FUNCTION_BLOCK FB_EL5131_SingleCycle
VAR_INPUT PERSISTENT
	arDataSingle											:	ARRAY[1..2] OF ST_EL5131_CamData;
END_VAR
VAR_INPUT
	bSetCounter												:	BOOL;
	nSetCounterValue										:	UDINT;
	bReset													:	BOOL;
	bRun													:	BOOL;
	stEl5131												:	REFERENCE TO ST_EL5131;
END_VAR
VAR_OUTPUT
	bInited													:	BOOL;
END_VAR
VAR
	{attribute 'hide'}
	_bLastCounterValue										:	BOOL;
	{attribute 'hide'}
	nLastCounterValue										:	UDINT;
	{attribute 'hide'}
	bForward												:	BOOL;
	{attribute 'hide'}
	bBackward												:	BOOL;
	{attribute 'hide'}
	rtSetCounter											:	R_TRIG;
END_VAR


// check REFERENCE
IF NOT __ISVALIDREF(stEl5131)
THEN 
	RETURN;
END_IF

// reset
IF bReset THEN 
	stEl5131.PlcToPdo.Contro_OutputChn1.Control.Enable_thresholds_output		:= FALSE;
	bReset 																		:= FALSE;	
	bInited																		:= FALSE;
END_IF

// init
IF NOT bInited THEN 
	stEl5131.PlcToPdo.Contro_OutputChn1.Control.Enable_thresholds_output		:= TRUE;
	stEl5131.PlcToPdo.Contro_OutputChn1.Control.Disalbe_thresholds_ccw			:= TRUE; // 在RUN 中根据情况再给false
	stEl5131.PlcToPdo.Contro_OutputChn1.Control.Disalbe_thresholds_cw			:= TRUE; // 在RUN 中根据情况再给false
	stEl5131.PlcToPdo.Contro_OutputChn1.Control.Set_tristate					:= FALSE;
	bInited																		:= TRUE;
END_IF

// set counter // 设置完成信号 stEl5131.PdoToPlc.Status.Set_counter_done
rtSetCounter(CLK:= bSetCounter, Q=> );
IF rtSetCounter.Q THEN 
	stEl5131.PlcToPdo.Set_counter_value				:= nSetCounterValue;	
	stEl5131.PlcToPdo.Control.Set_counter			:= TRUE;
END_IF
IF stEl5131.PdoToPlc.Status.Set_counter_done THEN 
	stEl5131.PlcToPdo.Control.Set_counter		:= FALSE;
END_IF
	
// run 启动位置比较输出功能，改例程只用两个位置点
IF bRun THEN 
	stEl5131.PlcToPdo.Contro_OutputChn1.Output_state.0 	:= TRUE;
	stEl5131.PlcToPdo.Contro_OutputChn1.Threshold[1] 	:= 600;// 脉冲
	stEl5131.PlcToPdo.Contro_OutputChn1.Duration[1]		:= 0;
	
	stEl5131.PlcToPdo.Contro_OutputChn1.Output_state.1 	:= FALSE;
	stEl5131.PlcToPdo.Contro_OutputChn1.Threshold[2] 	:= 1000;
	stEl5131.PlcToPdo.Contro_OutputChn1.Duration[2]		:= 0;
	
	stEl5131.PlcToPdo.Contro_OutputChn1.Control.Disalbe_thresholds_ccw	:= TRUE;// 正向
	stEl5131.PlcToPdo.Contro_OutputChn1.Control.Disalbe_thresholds_cw	:= FALSE;
	stEl5131.PlcToPdo.Contro_OutputChn1.Number_of_output_events := 2;
END_IF

END_FUNCTION_BLOCK
